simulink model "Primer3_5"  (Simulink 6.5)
settings: Solver=ode23t  SolverMode=SingleTasking  StartTime=0.0  StopTime=0  RelTol=1e-3  AbsTol=1e-6
undefined symbols (not defined in the file or in its folder): Phasor, powergui, steady, ZData
libraries: powerlib x22

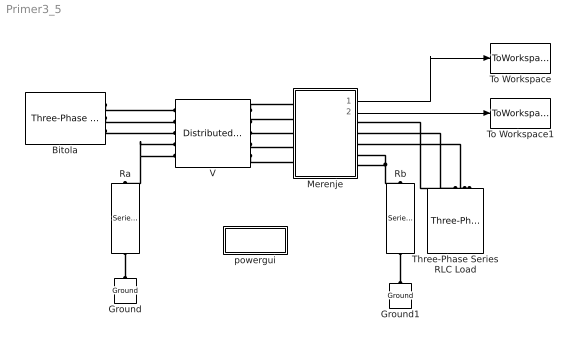
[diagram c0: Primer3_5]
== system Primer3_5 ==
  Bitola : powerlib/Electrical Sources/Three-Phase Source  DialogController=PMDialogs.PMDefaultMaskDlg  SystemSampleTime=-1  Voltage=410e3  PhaseAngle=0  Frequency=50  InternalConnection=Yg  SpecifyImpedance=on  Resistance=0.8929  Inductance=16.58e-3  ShortCircuitLevel=sqrt(3)*400e3*16e3  BaseVoltage=400e3  XRratio=10
  Ground : powerlib/Elements/Ground  Orientation=down  DialogController=PMDialogs.PMDefaultMaskDlg  PhysicalDomain=powersysdomain  SubClassName=unknown  LeftPortType=p1  RightPortType=p1  LConnTagsString=a
  Ground1 : powerlib/Elements/Ground  Orientation=down  DialogController=PMDialogs.PMDefaultMaskDlg  PhysicalDomain=powersysdomain  SubClassName=unknown  LeftPortType=p1  RightPortType=p1  LConnTagsString=a
  Merenje : Subsystem
  Ra : powerlib/Elements/Series RLC Branch  Orientation=down  DialogController=PMDialogs.PMDefaultMaskDlg  PhysicalDomain=powersysdomain  SubClassName=unknown  LeftPortType=p1  RightPortType=p1  LConnTagsString=__new0  RConnTagsString=__new0  BranchType=R  Resistance=0.5  Inductance=1e-3  SetiL0=off  InitialCurrent=0  Capacitance=1e-6  Setx0=off  InitialVoltage=0  Measurements=None
  Rb : powerlib/Elements/Series RLC Branch  Orientation=down  DialogController=PMDialogs.PMDefaultMaskDlg  PhysicalDomain=powersysdomain  SubClassName=unknown  LeftPortType=p1  RightPortType=p1  LConnTagsString=__new0  RConnTagsString=__new0  BranchType=R  Resistance=0.5  Inductance=1e-3  SetiL0=off  InitialCurrent=0  Capacitance=1e-6  Setx0=off  InitialVoltage=0  Measurements=None
  Three-Phase Series RLC Load : powerlib/Elements/Three-Phase Series RLC Load  Orientation=down  DialogController=PMDialogs.PMDefaultMaskDlg  PhysicalDomain=powersysdomain  SubClassName=unknown  LeftPortType=p1  RightPortType=p1  LConnTagsString=A|B|C  Configuration=Y (grounded)  NominalVoltage=400e3  NominalFrequency=50  ActivePower=1000e6  InductivePower=0  CapacitivePower=0  Measurements=None
  To Workspace : ToWorkspace  VariableName=napon  SampleTime=-1  SaveFormat=Array
  To Workspace1 : ToWorkspace  VariableName=struja  SampleTime=-1  SaveFormat=Array
  V : powerlib/Elements/Distributed Parameters Line  DialogController=PMDialogs.PMDefaultMaskDlg  SystemSampleTime=-1  Phases=5  Frequency=50  Resistance=[0.077552 0.048545 0.048526 0.04828 0.048266;0.048545 0.077556 0.048545 0.04828 0.04828;0.048526 0.048545 0.077552 0.048266 0.04828;0.04828 0.04828 0.048266 0.66802 0.048008;0.048266 0.04828 0.04828 0.048008 0.66802]  Inductance=[0.0019739 0.0010122 0.00087354 0.0010299 0.00089553;0.0010122 0.0019739 0.0010122 0.0010089 0.0010089;0.00087354 0.0010122 0.0019739 0.00089553 0.0010299;0.0010299 0.0010089 0.00089553 0.0024807 0.00097794;0.00089553 0.0010089 0.0010299 0.00097794 0.0024807]  Capacitance=[1.0643e-008 -1.3918e-009 -3.4639e-010 -1.2909e-009 -4.2739e-010;-1.3918e-009 1.0936e-008 -1.3918e-009 -1.0228e-009 -1.0228e-009;-3.4639e-010 -1.3918e-009 1.0643e-008 -4.2739e-010 -1.2909e-009;-1.2909e-009 -1.0228e-009 -4.2739e-010 7.0383e-009 -7.334e-010;-4.2739e-010 -1.0228e-009 -1.2909e-009 -7.334e-010 7.0383e-009]  Length=113.5  x1=[0 15403.3627837788 -263615.643386196 -307282.21591848 4195.39995859801 -31105.74577435;0.000130826521382094 16042.4660984549 -250815.522307551 -317862.318848337 4335.73983084752 -29588.5378209512;0.000261653042764188 16654.4736537612 -237591.773278133 -327905.551645424 4468.75662929868 -28021.3547642249;0.000392479564146282 17238.3517676348 -223966.731238185 -337394.951268182 4594.22568829593 -26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  x2=[0 14355.18102281 -306480.27836917 -259068.878686489 2493.08147836403 -36192.6929974387;0.000130826521382094 15097.7703913987 -296041.908140833 -271220.317826871 2643.10913545235 -34954.4140711386;0.000261653042764188 15814.8595936766 -285103.522499833 -282913.665273436 2788.67257558782 -33657.0970651088;0.000392479564146282 16505.2374644555 -273683.596402788 -294129.170937471 2929.52594181037 -32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  x3=[0 1.00955054864897 499.700119190369 203.757483344405 -9.71002584490683 -67.4763134179193;0.000130826521382094 1.68129649276911 486.947567132447 216.221674115035 -9.95805184057227 -68.2659422107709;0.000261653042764188 2.35020272353611 473.372559597684 228.320666018086 -10.1892586654938 -68.9402696819965;0.000392479564146282 3.01513945690312 458.998024802686 240.034023830492 -10.4032558108522 -69.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  x4="[0 28.5295818869429 -2384.24813674944 -2157.25552420489 24.4937740921161 -79.4564214710984;0.000130826521382094 29.5627121194917 -2303.47455925964 -2258.46990440231 25.4718093635823 -73.3515782016976;0.000261653042764188 30.5459108683778 -2218.81040833874 -2355.86972412643 26.4068226948436 -67.1228439606628;0.000392479564146282 31.4775175088223 -2130.39868191775 -2449.29047487451 27.2972348463942 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"  x5=0.00065413260691047  Measurements=None
  powergui : Subsystem  AncestorBlock=powerlib/powergui  InitFcn=powergui( 'InitFcn_Callback' , gcb , 0 , [ ] );  mask(PSB option menu block){SimulationMode=Phasor, SampleTime=50e-6, echomessages=off, RestoreLinks=warning, x0status=steady, Frange=[0:2:500], Ylog=off, Xlog=on, ShowGrid=off, save=off, variable=ZData, structure=, ZoomFFT=on, StartTime=0.0, cycles=1, DisplayStyle=1, fundamental=60, FreqAxis=off, MaxFrequency=1000, frequencyindice=50, frequencyindicesteady=1, RmsSteady=2, display=off, Ts=0, frequency=50, methode=off, HookPort=off, Interpol=off}
      mask prompts: SimulationMode "Simulation mode"; SampleTime "Sample time Ts (when simulation mode is Discrete) (s)"; echomessages "Echo  Messages"; RestoreLinks "Restore disabled links"; x0status "Initial electrical states status"; Frange "Impedance tool: Frequency Range"; Ylog "Impedance tool: Log impedance"; Xlog "Impedance tool: log Frequency"; ShowGrid "Impedance tool: grid"; save "Impedance tool: Save Data To Workspace"; variable "Impedance tool: Variable Name"; structure "Structure Name (PSBFFTSCOPE)"; ZoomFFT "ZoomFFT (PSBFFTSCOPE)"; StartTime "Start Time (PSBFFTSCOPE)"; cycles "Cycles (PSBFFTSCOPE)"; DisplayStyle "Display style (PSBFFTSCOPE)"; fundamental "Fundamental (PSBFFTSCOPE)"; FreqAxis "Frequency Axis (PSBFFTSCOPE)"; MaxFrequency "Max Frequency (PSBFFTSCOPE)"; frequencyindice "Load flow frequency (Hz)"; frequencyindicesteady "Frequency indice (STEADYSTATE)"; RmsSteady "RMS display (STEADYSTATE)"; display "Display Results"; Ts "OBSOLETE 1"; frequency "Phasor frequency (Hz)"; methode "Phasor simulation"; HookPort "Hook port"; Interpol "Interpolate"
      mask init:
      | powerlibroot = which('powersysdomain');
      | PSBroot = powerlibroot(1:end-16);
      | %
      | switch SimulationMode
      | 	case 1
      | 		message=sprintf('Continuous');
      | 	case 2
      |         SampleTimeeval=evalin('base',SampleTime,'NaN');
      |         if isnan(SampleTimeeval)
      |             message=sprintf('Warning !!,\nUndefined sample time');
      |         else
      |             message=sprintf('Discrete,\nTs = %.4g s.',SampleTimeeval);
      |         end
      | 	case 3
      | 		message=sprintf('Phasors');
      | end
      | if strcmp(bdroot,'powerlib')
      |   message='powergui';
      | end
      | power_initmask();
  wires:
  Merenje/2(I) -> To Workspace1/1
  Merenje/1(U) -> To Workspace/1
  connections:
  Ground/LConn1 -- Ra/RConn1
  Ground1/LConn1 -- Rb/RConn1
  V/RConn1 -- Merenje/LConn1
  V/RConn2 -- Merenje/LConn2
  V/RConn3 -- Merenje/LConn3
  V/RConn4 -- Merenje/LConn4
  V/RConn5 -- Merenje/LConn5
  Merenje/RConn4 -- Rb/LConn1 -- Merenje/RConn5
  Merenje/RConn1 -- Three-Phase Series RLC Load/LConn1
  Merenje/RConn2 -- Three-Phase Series RLC Load/LConn2
  Merenje/RConn3 -- Three-Phase Series RLC Load/LConn3
  Bitola/RConn1 -- V/LConn1
  Bitola/RConn2 -- V/LConn2
  Bitola/RConn3 -- V/LConn3
  V/LConn5 -- Ra/LConn1 -- V/LConn4

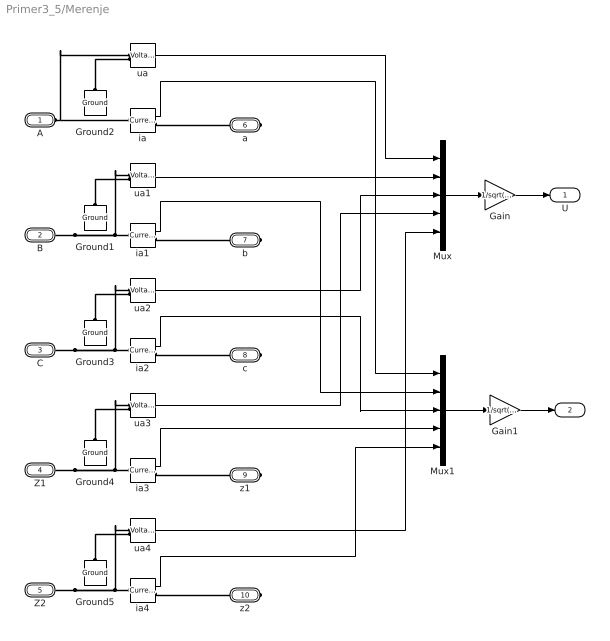
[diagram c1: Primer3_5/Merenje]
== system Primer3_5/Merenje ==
  Gain : Gain  Gain=1/sqrt(2)
  Gain1 : Gain  Gain=1/sqrt(2)
  Ground{1..5} (5 alike) : powerlib/Elements/Ground  Orientation=down  DialogController=PMDialogs.PMDefaultMaskDlg  PhysicalDomain=powersysdomain  SubClassName=unknown  LeftPortType=p1  RightPortType=p1  LConnTagsString=a
  Mux : Mux  Inputs=5
  Mux1 : Mux  Inputs=5
  ia{,1..4} (5 alike) : powerlib/Measurements/Current Measurement  DialogController=PMDialogs.PMDefaultMaskDlg  SystemSampleTime=-1  PhasorSimulation=on  OutputType=Complex  PSBequivalent=0
  ua{,1..4} (5 alike) : powerlib/Measurements/Voltage Measurement  DialogController=PMDialogs.PMDefaultMaskDlg  SystemSampleTime=-1  PhasorSimulation=on  OutputType=Complex  PSBequivalent=0
  A : PMIOPort  Port=1  Side=Left
  B : PMIOPort  Port=2  Side=Left
  C : PMIOPort  Port=3  Side=Left
  Z1 : PMIOPort  Port=4  Side=Left
  Z2 : PMIOPort  Port=5  Side=Left
  a : PMIOPort  Orientation=left  Port=6  Side=Right
  b : PMIOPort  Orientation=left  Port=7  Side=Right
  c : PMIOPort  Orientation=left  Port=8  Side=Right
  z1 : PMIOPort  Orientation=left  Port=9  Side=Right
  z2 : PMIOPort  Orientation=left  Port=10  Side=Right
  U : Outport
  I : Outport  Port=2
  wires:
  ua/1 -> Mux/1
  ia/1 -> Mux1/1
  ua1/1 -> Mux/2
  ia1/1 -> Mux1/2
  ua2/1 -> Mux/3
  ia2/1 -> Mux1/3
  ua3/1 -> Mux/4
  ia3/1 -> Mux1/4
  ua4/1 -> Mux/5
  ia4/1 -> Mux1/5
  Mux/1 -> Gain/1
  Gain/1 -> U/1
  Mux1/1 -> Gain1/1
  Gain1/1 -> I/1
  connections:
  A/RConn1 -- ia/LConn1 -- ua/LConn1
  ia/RConn1 -- a/RConn1
  Ground2/LConn1 -- ua/LConn2
  ia1/LConn1 -- B/RConn1 -- ua1/LConn1
  Ground1/LConn1 -- ua1/LConn2
  ia1/RConn1 -- b/RConn1
  ia2/LConn1 -- ua2/LConn1 -- C/RConn1
  ia2/RConn1 -- c/RConn1
  Ground3/LConn1 -- ua2/LConn2
  ia3/LConn1 -- Z1/RConn1 -- ua3/LConn1
  Ground4/LConn1 -- ua3/LConn2
  ia3/RConn1 -- z1/RConn1
  ia4/LConn1 -- ua4/LConn1 -- Z2/RConn1
  Ground5/LConn1 -- ua4/LConn2
  ia4/RConn1 -- z2/RConn1

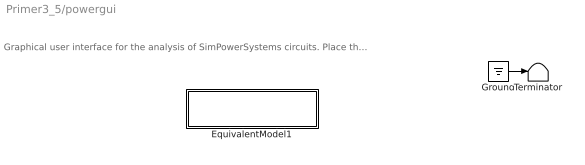
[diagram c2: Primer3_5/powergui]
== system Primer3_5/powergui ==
  note: Graphical user interface for the analysis of SimPowerSystems circuits. Place the Powergui block in the top-level of your model and double-click on it to open the GUI.
  EquivalentModel1 : Subsystem
  Ground : Ground
  Terminator : Terminator
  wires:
  Ground/1 -> Terminator/1

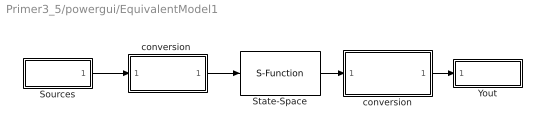
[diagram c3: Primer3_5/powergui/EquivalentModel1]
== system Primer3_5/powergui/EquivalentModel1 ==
  Sources : Subsystem
  State-Space : S-Function  FunctionName=sfun_psbdqc  Parameters=H, Rswitch,InputsNonZero
  Yout : Subsystem
  conversion : Subsystem
  "conversion " : Subsystem
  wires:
  State-Space/1 -> conversion/1(Yout)
  conversion/1(Complex) -> Yout/1(v,i)
  "conversion "/1(u) -> State-Space/1
  Sources/1(u) -> "conversion "/1(Complex)

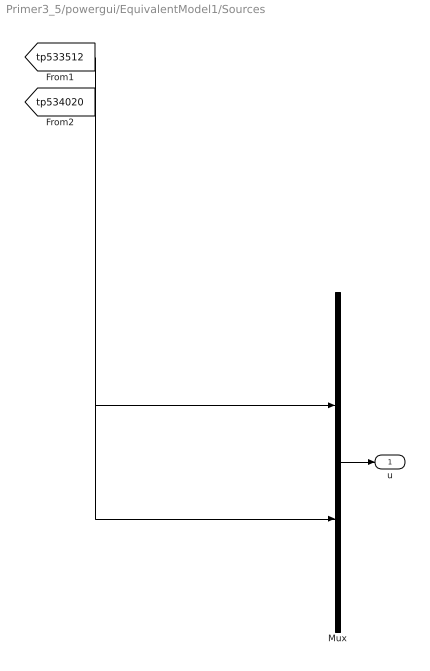
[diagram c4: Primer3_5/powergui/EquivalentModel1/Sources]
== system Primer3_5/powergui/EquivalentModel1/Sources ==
  Mux : Mux  Inputs=[10 3]
  u : Outport
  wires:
  Mux/1 -> u/1
  [tp533512] -> Mux/1
  [tp534020] -> Mux/2

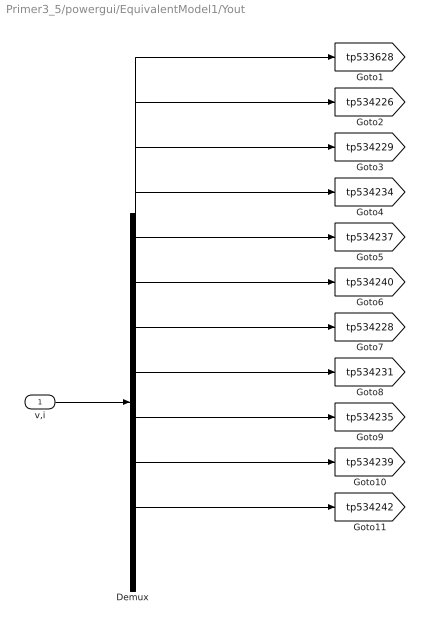
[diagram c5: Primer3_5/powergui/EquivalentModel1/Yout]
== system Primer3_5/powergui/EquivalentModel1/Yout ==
  v,i : Inport
  Demux : Demux  Outputs=[10 1 1 1 1 1 1 1 1 1 1]
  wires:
  v,i/1 -> Demux/1
  Demux/1 -> [tp533628]
  Demux/2 -> [tp534226]
  Demux/3 -> [tp534229]
  Demux/4 -> [tp534234]
  Demux/5 -> [tp534237]
  Demux/6 -> [tp534240]
  Demux/7 -> [tp534228]
  Demux/8 -> [tp534231]
  Demux/9 -> [tp534235]
  Demux/10 -> [tp534239]
  Demux/11 -> [tp534242]

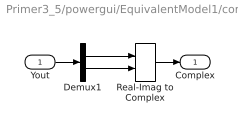
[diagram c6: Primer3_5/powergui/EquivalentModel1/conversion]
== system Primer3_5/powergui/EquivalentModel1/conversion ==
  Yout : Inport
  Demux1 : Demux  Outputs=2
  Real-Imag to Complex : RealImagToComplex
  Complex : Outport
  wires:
  Demux1/1 -> Real-Imag to Complex/1
  Demux1/2 -> Real-Imag to Complex/2
  Real-Imag to Complex/1 -> Complex/1
  Yout/1 -> Demux1/1

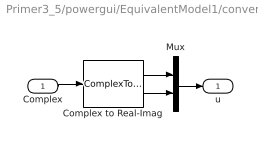
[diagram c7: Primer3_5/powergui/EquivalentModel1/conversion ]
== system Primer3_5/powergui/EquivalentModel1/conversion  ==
  Complex : Inport
  Complex to Real-Imag : ComplexToRealImag
  Mux : Mux  Inputs=2
  u : Outport
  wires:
  Complex to Real-Imag/1 -> Mux/1
  Complex to Real-Imag/2 -> Mux/2
  Complex/1 -> Complex to Real-Imag/1
  Mux/1 -> u/1
